// ------------------------------------------------------------------
// File           : C:\Users\acer\Documents\190.awl
//
// Source File    : C:\Users\acer\Documents\190.var
// Generation Date: 6/21/2019  Time: 3:19:16 PM
// ------------------------------------------------------------------

DATA_BLOCK DB  190
VERSION : 0.0


STRUCT

 V1_M_r0027_27:
   STRUCT
   SYNTAX_ID : BYTE := B#16#82;
   bereich_u_einheit : BYTE := B#16#A1;
   spalte : WORD := W#16#1B;
   zeile : WORD := W#16#1;
   bausteintyp : BYTE := B#16#1A;
   ZEILENANZAHL : BYTE := B#16#1;
   typ : BYTE := B#16#8;
   laenge : BYTE := B#16#4;
   END_STRUCT ;

 V2_M_r0027_27:
   STRUCT
   SYNTAX_ID : BYTE := B#16#82;
   bereich_u_einheit : BYTE := B#16#A2;
   spalte : WORD := W#16#1B;
   zeile : WORD := W#16#1;
   bausteintyp : BYTE := B#16#1A;
   ZEILENANZAHL : BYTE := B#16#1;
   typ : BYTE := B#16#8;
   laenge : BYTE := B#16#4;
   END_STRUCT ;

 V3_M_r0027_27:
   STRUCT
   SYNTAX_ID : BYTE := B#16#82;
   bereich_u_einheit : BYTE := B#16#A3;
   spalte : WORD := W#16#1B;
   zeile : WORD := W#16#1;
   bausteintyp : BYTE := B#16#1A;
   ZEILENANZAHL : BYTE := B#16#1;
   typ : BYTE := B#16#8;
   laenge : BYTE := B#16#4;
   END_STRUCT ;

 V4_M_r0027_27:
   STRUCT
   SYNTAX_ID : BYTE := B#16#82;
   bereich_u_einheit : BYTE := B#16#A4;
   spalte : WORD := W#16#1B;
   zeile : WORD := W#16#1;
   bausteintyp : BYTE := B#16#1A;
   ZEILENANZAHL : BYTE := B#16#1;
   typ : BYTE := B#16#8;
   laenge : BYTE := B#16#4;
   END_STRUCT ;

 V5_M_r0027_27:
   STRUCT
   SYNTAX_ID : BYTE := B#16#82;
   bereich_u_einheit : BYTE := B#16#A5;
   spalte : WORD := W#16#1B;
   zeile : WORD := W#16#1;
   bausteintyp : BYTE := B#16#1A;
   ZEILENANZAHL : BYTE := B#16#1;
   typ : BYTE := B#16#8;
   laenge : BYTE := B#16#4;
   END_STRUCT ;

 END_STRUCT ;

BEGIN
END_DATA_BLOCK
